(* Logix 5000 AddOnInstructionDefinition export AMCI_SD4840E2_Jog_CCW; software revision 20.03 *)

ADD_ON_INSTRUCTION AMCI_SD4840E2_Jog_CCW   (* revision 5.0, vendor AMCI, ExecuteEnableInFalse *)
// Revision note:
// Version 5.0 added the (hidden) ability to program the motor current and unlatched the error bit if the rung goes false.
VAR_INPUT
   Axis_Status_Bits : INT; {required}
   Programmed_Speed : DINT; {required}
   Acceleration : INT; {required}
   Deceleration : INT; {required}
   motor_current : INT;
   Jerk : INT;
END_VAR
VAR_OUTPUT
   EN : BOOL; {access Read Only, visible}
   Jog_CCW_Occurring : BOOL; {access Read Only, visible}
END_VAR
VAR_IN_OUT
   AMCI_SD4840E2_output_data : _000A:SD4840E2_4342D302:O:0; {required}
END_VAR
VAR_OUTPUT
   ER : BOOL; {access Read Only, visible}
END_VAR
VAR
   Upper_Result_X_1000 : DINT;
   command_data_block : INT[10];
        [0]   // Command Bits MSW
        [1]   // Command Bits LSW
        [2]   // Upper Target Position
        [3]   // Lower Target Position
        [4]   // Upper Programmed Speed
        [5]   // Lower Programmed Speed
END_VAR

ROUTINE EnableInFalse   (* ladder *)
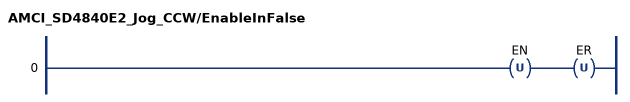
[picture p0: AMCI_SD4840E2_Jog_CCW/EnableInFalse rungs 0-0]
   0: OTU(EN)OTU(ER);
END_ROUTINE

ROUTINE Logic   (* ladder *)
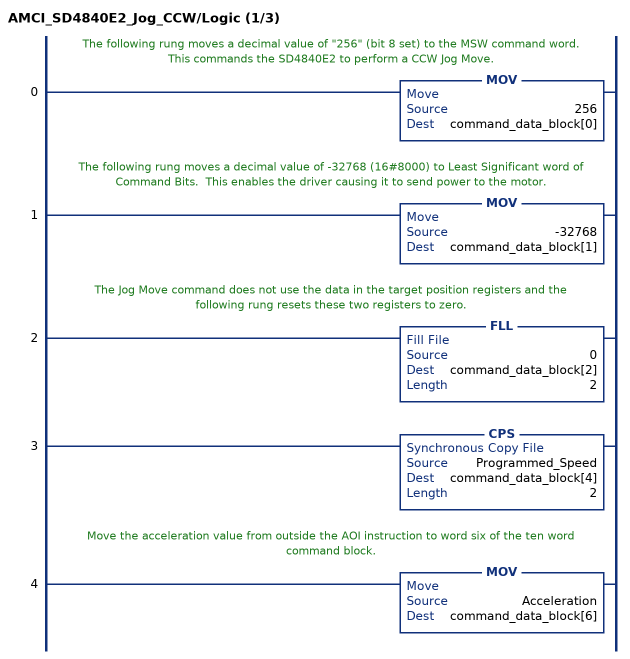
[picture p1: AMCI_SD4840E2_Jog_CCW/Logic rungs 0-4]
   // The following rung moves a decimal value of "256" (bit 8 set) to the MSW command word.  This commands the SD4840E2 to perform a CCW Jog Move.
   0: MOV(256,command_data_block[0]);
   // The following rung moves a decimal value of -32768 (16#8000) to Least Significant word of Command Bits.  This enables the driver causing it to send power to the motor.
   1: MOV(-32768,command_data_block[1]);
   // The Jog Move command does not use the data in the target position registers and the following rung resets these two registers to zero.
   2: FLL(0,command_data_block[2],2);
   3: CPS(Programmed_Speed,command_data_block[4],2);
   // Move the acceleration value from outside the AOI instruction to word six of the ten word command block.
   4: MOV(Acceleration,command_data_block[6]);
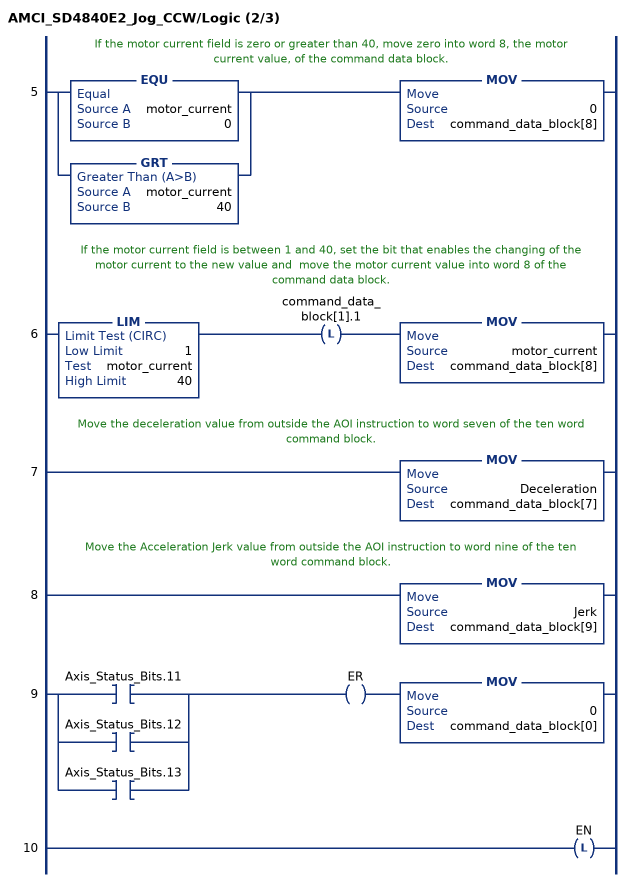
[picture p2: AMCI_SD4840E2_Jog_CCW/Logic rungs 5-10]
   // If the motor current field is zero or greater than 40, move zero into word 8, the motor current value, of the command data block.
   5: [EQU(motor_current,0) ,GRT(motor_current,40) ]MOV(0,command_data_block[8]);
   // If the motor current field is between 1 and 40, set the bit that enables the changing of the motor current to the new value and  move the motor current value into word 8 of the command data block.
   6: LIM(1,motor_current,40)OTL(command_data_block[1].1)MOV(motor_current,command_data_block[8]);
   // Move the deceleration value from outside the AOI instruction to word seven of the ten word command block.
   7: MOV(Deceleration,command_data_block[7]);
   // Move the Acceleration Jerk value from outside the AOI instruction to word nine of the ten word command block.
   8: MOV(Jerk,command_data_block[9]);
   9: [XIC(Axis_Status_Bits.11) ,XIC(Axis_Status_Bits.12) ,XIC(Axis_Status_Bits.13) ]OTE(ER)MOV(0,command_data_block[0]);
   10: OTL(EN);
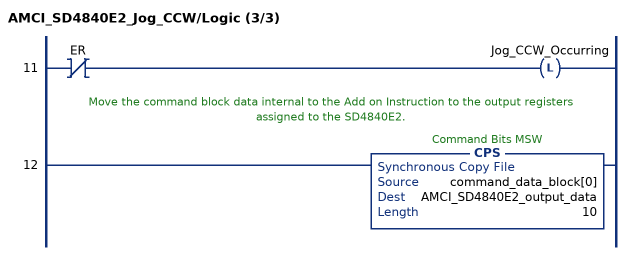
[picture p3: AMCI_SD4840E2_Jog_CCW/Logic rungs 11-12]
   11: XIO(ER)OTL(Jog_CCW_Occurring);
   // Move the command block data internal to the Add on Instruction to the output registers assigned to the SD4840E2.
   12: CPS(command_data_block[0],AMCI_SD4840E2_output_data,10);
END_ROUTINE
END_ADD_ON_INSTRUCTION
